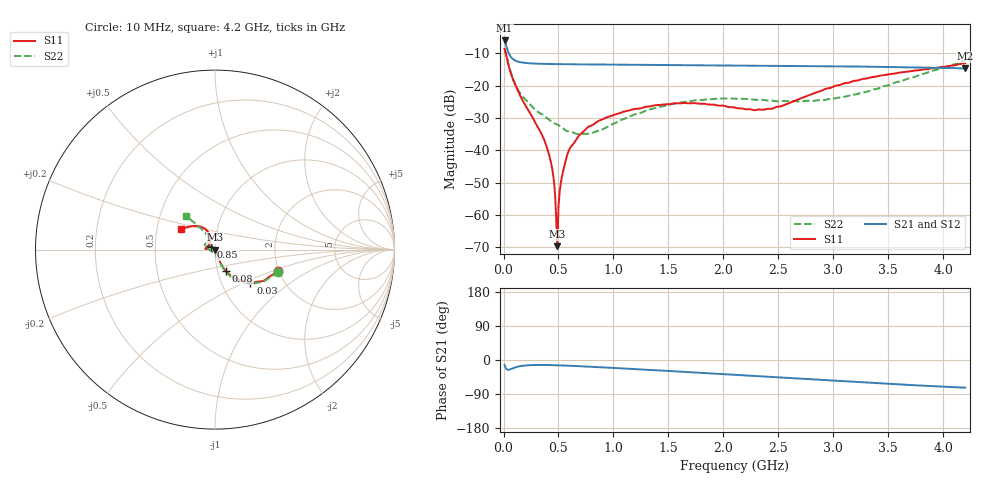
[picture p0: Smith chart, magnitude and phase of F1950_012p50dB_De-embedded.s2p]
! Integrated Device Technology
! Corporate Headquarters
! 6024 Silver Creek Valley Road
! San Jose, CA 95138  USA
! Phone:  1-408-284-8200
! Toll Free:  1-800-223-1366
! Webpage:  http://www.idt.com/
! Timing and RF Division
! 515 Groton Road, Suite 102
! Westford, MA 01886-6024
! Device:  F1950
! Description: 7-bit 0.25 dB Digital Step Attenuator
! Frequency:  150.0 -  4000.00 MHz
! Package:  4x4 mm Thin QFN Plastic Package: 24 pin
! Ports:  2 RF, 12 DC
!  Pin  1  = D0
!  Pin  2  = VDD
!  Pin  3  = Vmode
!  Pin  4  = GND
!  Pin  5  = RF1  =  Port 1
!  Pin  6  = GND
!  Pin  7  = GND
!  Pin  8  = GND
!  Pin  9  = GND
!  Pin 10  = GND
!  Pin 11  = GND
!  Pin 12  = GND
!  Pin 13  = GND
!  Pin 14  = RF2  =  Port 2
!  Pin 15  = GND
!  Pin 16  = LE
!  Pin 17  = CLK
!  Pin 18  = DATE
!  Pin 19  = D6
!  Pin 20  = D5
!  Pin 21  = D4
!  Pin 22  = D3
!  Pin 23  = D2
!  Pin 24  = D1
! State:  50
! Atten State:  12.50 dB
! Voltage:  +5.00 Volts
! Current:  Not Measured mA
! Data:  The device was measured on a the F195X evaluation board which has
!  individual transmission lines to the RF pins.  Data was collected
!  using a calibrated network analyzer.  The evaluation board was
!  de-embedded using a TRL calibration technique.
!  The reference plane is the edge of the package pin.
! Misc:  Board 2019
!  Action Tracker AT0250
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# GHz S dB R 50
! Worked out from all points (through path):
!   420 points, 10 MHz to 4.2 GHz, reference 50 ohm
!   highest |S21| = -5.99 dB at 10 MHz (marker M1); lowest = -14.7 dB at 4.2 GHz (marker M2)
!   group delay of S21, straight-line fit = 42.9 ps
!   lowest |S11| = -69.7 dB at 490 MHz (marker M3), VSWR 1.00, Z = 50 + j0.0278 ohm
!   |S11| at or under -10 dB: 20.83 MHz to end of sweep
!   |S22| runs from -35.0 to -8.5 dB; largest |S21 - S12| = 0.00031
!   S11 on the Smith chart (normalised r, x): 10 MHz: 1.99, -0.54; 30 MHz: 1.37, -0.54; 80 MHz: 1.10, -0.27; 850 MHz: 0.96, +0.03; 4.2 GHz: 0.66, +0.16
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0.01  -8.60 -18.6  -5.99 -13.5  -5.99 -13.5  -8.52 -19.5
0.03  -11.36 -43.0  -8.28 -24.8  -8.28 -24.8  -11.29 -44.4
0.08  -17.46 -63.1  -11.58 -22.3  -11.58 -22.3  -17.32 -63.8
0.18  -24.98 -66.7  -12.88 -15.0  -12.88 -15.0  -23.56 -71.9
0.39  -38.71 -58.4  -13.26 -13.2  -13.26 -13.2  -29.90 -79.5
0.44  -45.19 -57.9  -13.30 -13.5  -13.30 -13.5  -31.19 -83.5
0.45  -47.30 -56.7  -13.30 -13.6  -13.30 -13.6  -31.41 -84.8
0.47  -54.21 -51.7  -13.31 -13.8  -13.31 -13.8  -31.77 -87.6
0.49  -69.70 122.0  -13.32 -13.9  -13.32 -14.0  -32.06 -89.6
0.5  -57.60 131.9  -13.33 -14.0  -13.33 -14.1  -32.23 -90.2
0.53  -48.44 136.5  -13.34 -14.3  -13.34 -14.4  -32.92 -92.1
0.58  -41.39 133.5  -13.36 -14.9  -13.36 -14.9  -34.08 -101.0
0.71  -34.69 140.0  -13.40 -16.6  -13.40 -16.6  -34.96 -124.0
0.85  -31.21 145.9  -13.44 -18.6  -13.44 -18.7  -34.07 -150.0
1.1  -27.96 158.2  -13.52 -22.5  -13.52 -22.5  -30.23 -177.5
1.41  -25.99 170.2  -13.59 -27.5  -13.59 -27.5  -26.60 168.9
1.73  -25.39 176.8  -13.67 -32.7  -13.67 -32.8  -24.61 160.2
2.11  -26.85 169.1  -13.76 -39.2  -13.76 -39.3  -24.03 150.8
2.44  -27.15 136.6  -13.83 -44.8  -13.83 -44.8  -24.62 140.6
2.81  -22.57 112.2  -13.93 -51.2  -13.93 -51.2  -24.72 125.7
3.51  -16.43 122.0  -14.18 -63.1  -14.18 -63.1  -19.77 120.1
4.2  -13.01 148.6  -14.66 -72.9  -14.66 -73.0  -12.14 130.6
